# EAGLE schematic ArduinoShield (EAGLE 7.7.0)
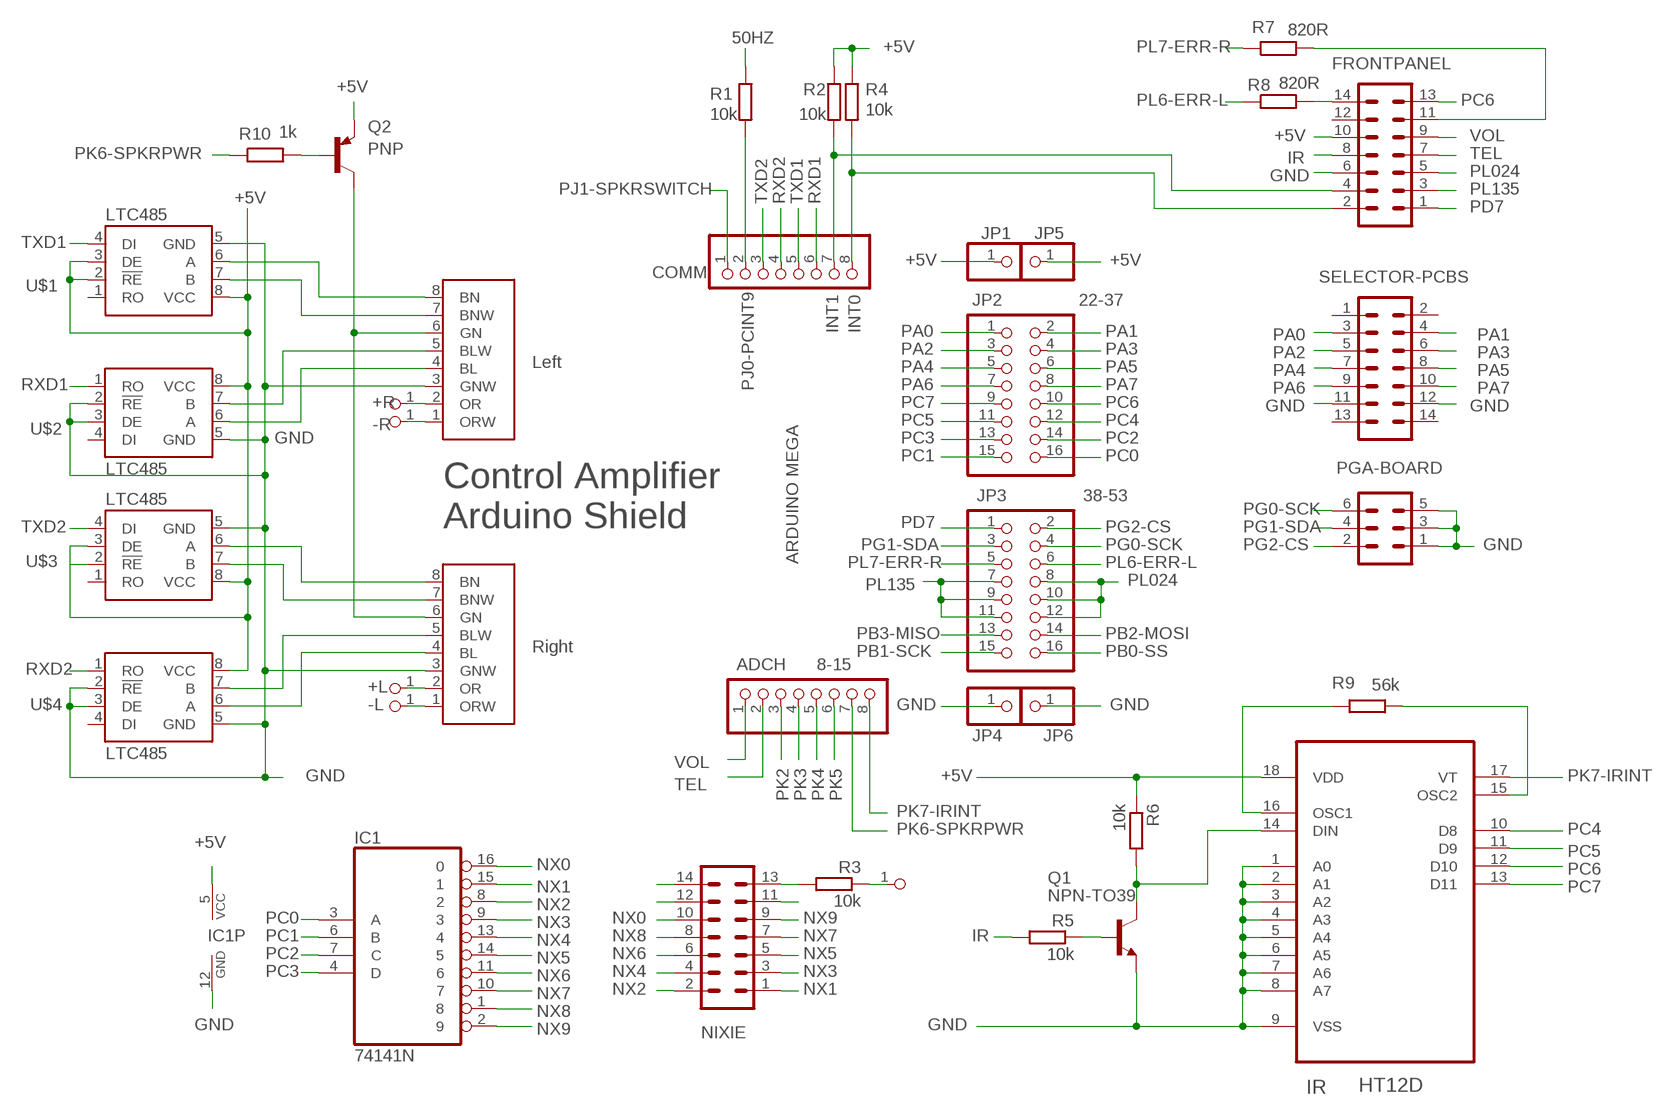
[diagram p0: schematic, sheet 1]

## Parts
+L  PINHDR-1X1  [HDR1X1]
+R  PINHDR-1X1  [HDR1X1]
-L  PINHDR-1X1  [HDR1X1]
-R  PINHDR-1X1  [HDR1X1]
ADCH  8-15  PINHD-1X8  [1X08]
COMM  PINHD-1X8  [1X08]
FRONTPANEL  PINHD-7X2  [MA07-2]
IC1  74141N  [DIL16]
IR  HT12D  [DIP254P762X342-18]
JP1  PINHD-1X1  [1X01]
JP2  22-37  PINHD-2X8  [2X08]
JP3  38-53  PINHD-2X8  [2X08]
JP4  PINHD-1X1  [1X01]
JP5  PINHD-1X1  [1X01]
JP6  PINHD-1X1  [1X01]
NIXIE  PINHD-7X2  [MA07-2]
PGA-BOARD  PINHD-3X2  [MA03-2]
Q1  NPN-TO39  [TO39]
Q2  PNP  PNP-TO39  [TO39]
R1  10k  R-EU_0207/10  [0207/10]
R2  10k  R-EU_0207/10  [0207/10]
R3  10k  R-EU_0207/10  [0207/10]
R4  10k  R-EU_0207/10  [0207/10]
R5  10k  R-EU_0207/10  [0207/10]
R6  10k  R-EU_0207/10  [0207/10]
R7  820R  R-EU_0207/10  [0207/10]
R8  820R  R-EU_0207/10  [0207/10]
R9  56k  R-EU_0207/10  [0207/10]
R10  1k  R-EU_0207/10  [0207/10]
SELECTOR-PCBS  PINHD-7X2  [MA07-2]
U$1  LTC485  [DIL08]
U$2  LTC485  [DIL08]
U$3  LTC485  [DIL08]
U$4  LTC485  [DIL08]
U$5  RJ45A  [1XRJ45_MM_JACK]
U$6  RJ45A  [1XRJ45_MM_JACK]
VNX  PINHDR-1X1  [HDR1X1]

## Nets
50HZ: R1.1
+5V: FRONTPANEL.10 IC1.5(VCC) IR.18(VDD) JP1.1 JP5.1 Q2.1(E) R2.1 R4.1 R6.1 U$1.2(!RE) U$1.3(DE) U$1.8(VCC) U$2.8(VCC) U$3.2(!RE) U$3.3(DE) U$3.8(VCC) U$4.8(VCC)
+L: -L.1 U$6.2(OR)
+R: +R.1 U$5.2(OR)
-L: +L.1 U$6.1(ORW)
-R: -R.1 U$5.1(ORW)
GND: FRONTPANEL.6 IC1.12(GND) IR.1(A0) IR.2(A1) IR.3(A2) IR.4(A3) IR.5(A4) IR.6(A5) IR.7(A6) IR.8(A7) IR.9(VSS) JP4.1 JP6.1 PGA-BOARD.1 PGA-BOARD.3 PGA-BOARD.5 Q1.1(E) SELECTOR-PCBS.11 SELECTOR-PCBS.12 U$1.5(GND) U$2.2(!RE) U$2.3(DE) U$2.5(GND) U$3.5(GND) U$4.2(!RE) U$4.3(DE) U$4.5(GND) U$5.3(GNW) U$6.3(GNW)
INT0: COMM.8 FRONTPANEL.2 R4.2
INT1: COMM.7 FRONTPANEL.4 R2.2
IR: FRONTPANEL.8 R5.2
N$1: R3.1 VNX.1
N$2: U$1.6(A) U$5.8(BN)
N$3: U$1.7(B) U$5.7(BNW)
N$4: U$2.6(A) U$5.4(BL)
N$5: IR.15(OSC2) R9.1
N$6: IR.14(DIN) Q1.3(C) R6.2
N$7: U$2.7(B) U$5.5(BLW)
N$9: FRONTPANEL.11 R7.2
N$10: IR.16(OSC1) R9.2
N$11: FRONTPANEL.14 R8.2
N$13: Q2.2(B) R10.2
N$14: Q1.2(B) R5.1
N$16: NIXIE.12
N$18: NIXIE.14
N$19: NIXIE.13 R3.2
N$20: U$3.6(A) U$6.8(BN)
N$21: NIXIE.11
N$22: U$3.7(B) U$6.7(BNW)
N$23: U$4.6(A) U$6.4(BL)
N$24: U$4.7(B) U$6.5(BLW)
N$100: Q2.3(C) U$5.6(GN) U$6.6(GN)
NX0: IC1.16 NIXIE.10
NX1: IC1.15 NIXIE.1
NX2: IC1.8 NIXIE.2
NX3: IC1.9 NIXIE.3
NX4: IC1.13 NIXIE.4
NX5: IC1.14 NIXIE.5
NX6: IC1.11 NIXIE.6
NX7: IC1.10 NIXIE.7
NX8: IC1.1 NIXIE.8
NX9: IC1.2 NIXIE.9
PA0: JP2.1 SELECTOR-PCBS.3
PA1: JP2.2 SELECTOR-PCBS.4
PA2: JP2.3 SELECTOR-PCBS.5
PA3: JP2.4 SELECTOR-PCBS.6
PA4: JP2.5 SELECTOR-PCBS.7
PA5: JP2.6 SELECTOR-PCBS.8
PA6: JP2.7 SELECTOR-PCBS.9
PA7: JP2.8 SELECTOR-PCBS.10
PB0-SS: JP3.16
PB1-SCK: JP3.15
PB2-MOSI: JP3.14
PB3-MISO: JP3.13
PC0: IC1.3(A) JP2.16
PC1: IC1.6(B) JP2.15
PC2: IC1.7(C) JP2.14
PC3: IC1.4(D) JP2.13
PC4: IR.10(D8) JP2.12
PC5: IR.11(D9) JP2.11
PC6: FRONTPANEL.13 IR.12(D10) JP2.10
PC7: IR.13(D11) JP2.9
PD7: FRONTPANEL.1 JP3.1
PG0-SCK: JP3.4 PGA-BOARD.6
PG1-SDA: JP3.3 PGA-BOARD.4
PG2-CS: JP3.2 PGA-BOARD.2
PJ0-PCINT9: COMM.2 R1.2
PJ1-SPKRSWITCH: COMM.1
PK2: ADCH.3
PK3: ADCH.4
PK4: ADCH.5
PK5: ADCH.6
PK6-SPKRPWR: ADCH.7 R10.1
PK7-IRINT: ADCH.8 IR.17(VT)
PL6-ERR-L: JP3.6 R8.1
PL7-ERR-R: JP3.5 R7.1
PL024: FRONTPANEL.5 JP3.8 JP3.10 JP3.12
PL135: FRONTPANEL.3 JP3.7 JP3.9 JP3.11
RXD1: COMM.6 U$2.1(RO)
RXD2: COMM.4 U$4.1(RO)
TEL: ADCH.2 FRONTPANEL.7
TXD1: COMM.5 U$1.4(DI)
TXD2: COMM.3 U$3.4(DI)
VOL: ADCH.1 FRONTPANEL.9
Unconnected: FRONTPANEL.12 SELECTOR-PCBS.1 SELECTOR-PCBS.2 SELECTOR-PCBS.13 SELECTOR-PCBS.14 U$1.1(RO) U$2.4(DI) U$3.1(RO) U$4.4(DI)

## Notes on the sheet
- Left
- Control Amplifier
  Arduino Shield
- ARDUINO MEGA
- Right

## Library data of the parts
+L +R -L -R VNX = Connector:PINHDR-1X1
ADCH COMM = pinhead:PINHD-1X8: PIN HEADER
FRONTPANEL NIXIE SELECTOR-PCBS = Header:PINHD-7X2: PIN HEADER
IC1 = IC_dig:74*141: BCD to decimal DECODER/DRIVER
IR = IC_dig:HT12D: Decoders; MPN: HT12D; OC_FARNELL: 1211514; OC_NEWARK: 24M2761; PACKAGE: DIP-18; SUPPLIER: HOLTEK
JP1 JP4-JP6 = pinhead:PINHD-1X1: PIN HEADER
JP2 JP3 = pinhead:PINHD-2X8: PIN HEADER
PGA-BOARD = Header:PINHD-3X2: PIN HEADER
Q1 = Trans:NPN: NPN Transistor
Q2 = Trans:PNP: PNP Transistror
R1-R10 = AJANLIB:R-EU_: RESISTOR, European symbol
U$1-U$4 = IC_Interface:LTC485: LTC485
U$5 U$6 = Connector:RJ45A

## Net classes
2 gnd: width 0.914 mm, drill 0.711 mm, clearance 0.305 mm
4 vcc2: width 0.914 mm, drill 0.305 mm, clearance 0.305 mm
